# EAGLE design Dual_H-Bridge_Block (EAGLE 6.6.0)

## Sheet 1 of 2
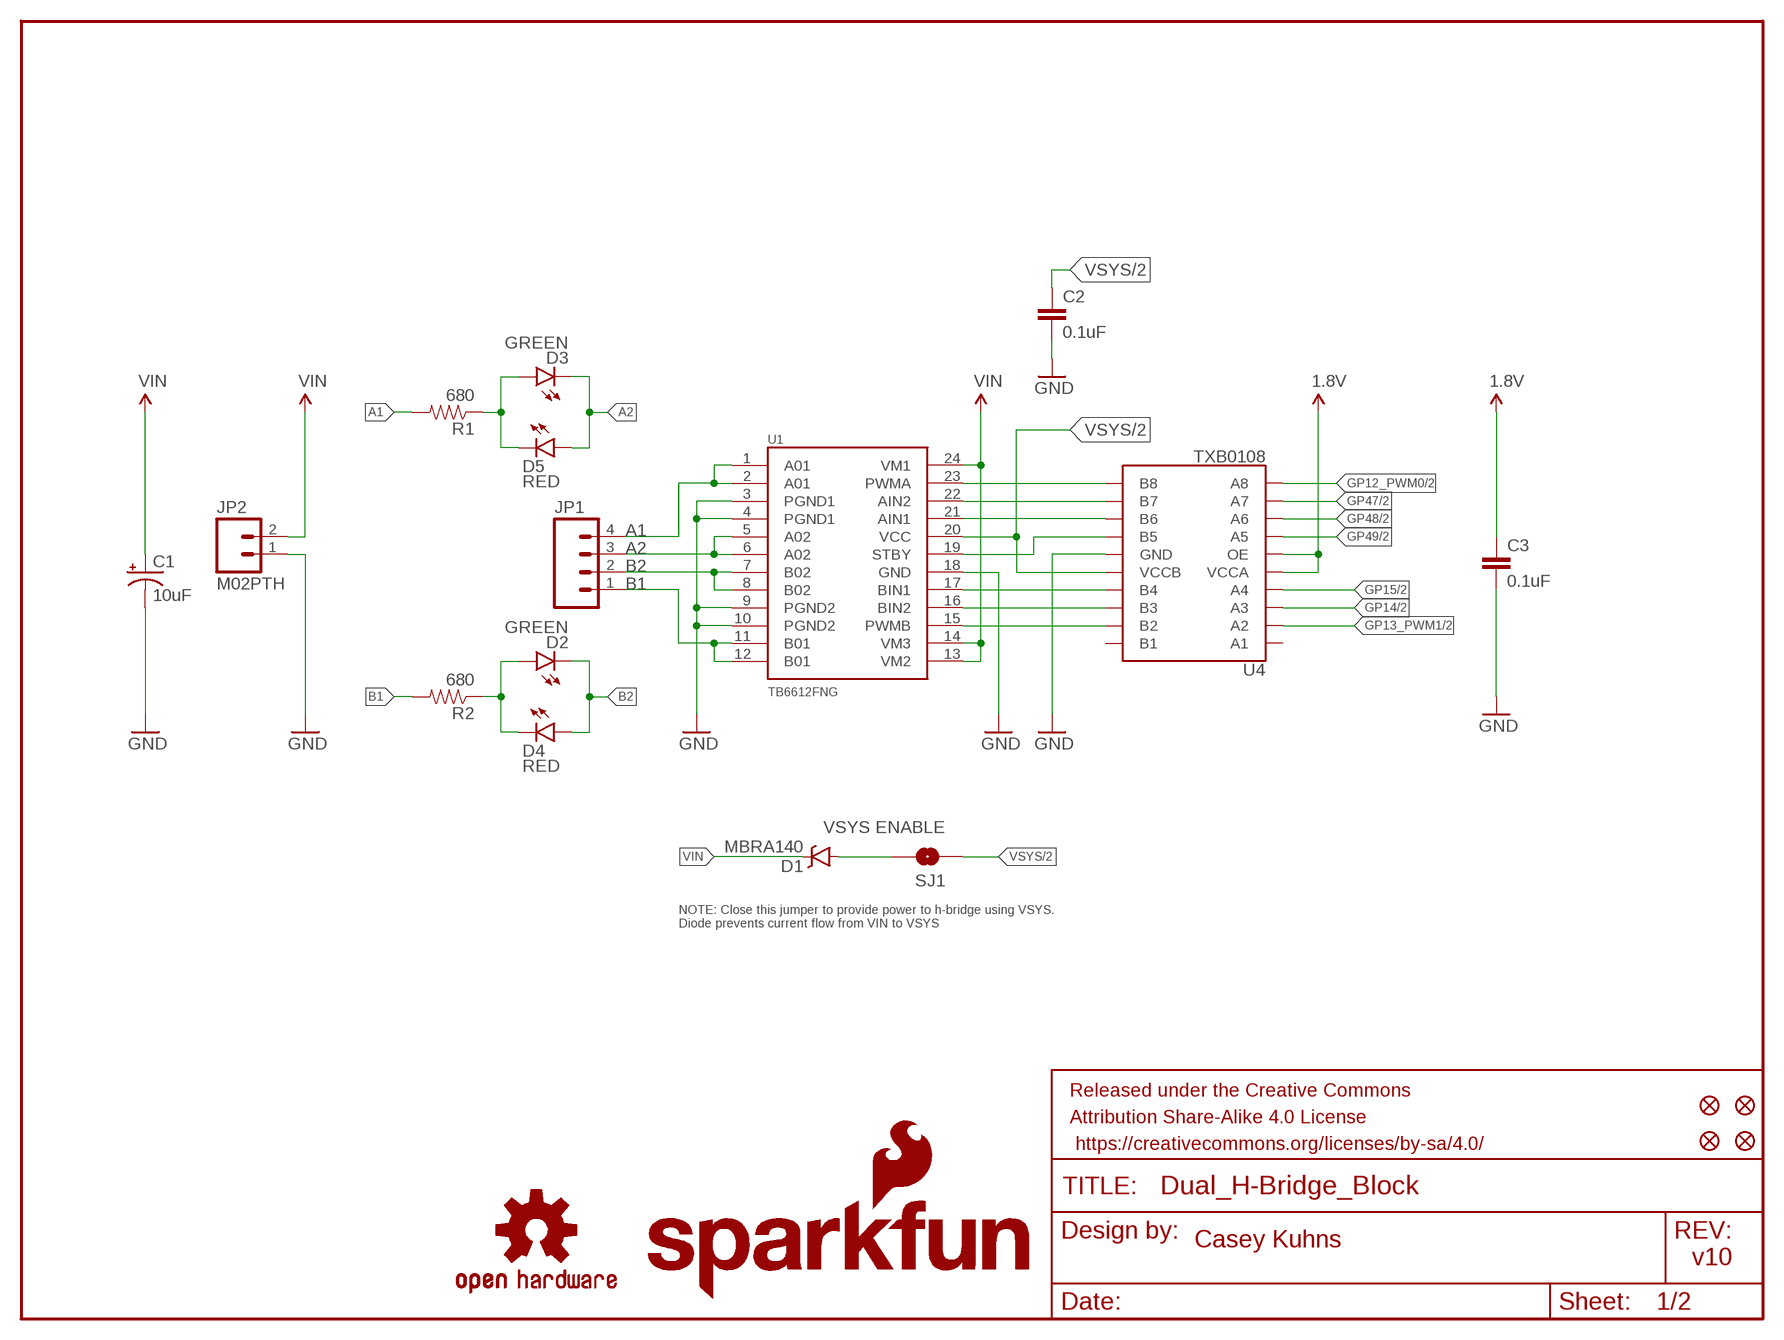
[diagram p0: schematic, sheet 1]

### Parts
C1  10uF  10UF-16V-10%(TANT)  [EIA3216]
C2  0.1uF  0.1UF-25V(+80/-20%)(0603)  [0603-CAP]
C3  0.1uF  0.1UF-25V(+80/-20%)(0603)  [0603-CAP]
D1  MBRA140  DIODE-SCHOTTKY-MBRA140  [SMA-DIODE]
D2  GREEN  LED-GREEN0603  [LED-0603]
D3  GREEN  LED-GREEN0603  [LED-0603]
D4  RED  LED-RED0603  [LED-0603]
D5  RED  LED-RED0603  [LED-0603]
FID1  FIDUCIAL1X2  [FIDUCIAL-1X2]
FID2  FIDUCIAL1X2  [FIDUCIAL-1X2]
FID3  FIDUCIAL1X2  [FIDUCIAL-1X2]
FID4  FIDUCIAL1X2  [FIDUCIAL-1X2]
FRAME1  FRAME-LETTER  [CREATIVE_COMMONS]
JP1  M04PTH  [1X04]
JP2  M02PTH  [1X02]
LOGO1  OSHW-LOGOS  [OSHW-LOGO-S]
LOGO4  SFE_LOGO_NAME_FLAME.1_INCH  [SFE_LOGO_NAME_FLAME_.1]
R1  680  680OHM1/10W5%(0603)  [0603-RES]
R2  680  680OHM1/10W5%(0603)  [0603-RES]
SJ1  VSYS ENABLE  JUMPER-PAD-2-NOYES_SILK  [PAD-JUMPER-2-NO_YES_SILK]
U1  TB6612FNG  TB6621FNG  [SSOP24]
U4  TXB0108  [UFDFN-20]

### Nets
1.8V: C3.1 U4.5(VCCA) U4.6(OE) ; also sheet 2
A1: JP1.4 R1.2 U1.1(A01) U1.2(A01)
A2: D3.C D5.A JP1.3 U1.5(A02) U1.6(A02)
B1: JP1.1 R2.2 U1.11(B01) U1.12(B01)
B2: D2.C D4.A JP1.2 U1.7(B02) U1.8(B02)
GND: C1.C(-) C2.2 C3.2 JP2.1 U1.3(PGND1) U1.4(PGND1) U1.9(PGND2) U1.10(PGND2) U1.18(GND) U4.15(GND) ; also sheet 2
GP12_PWM0: U4.10(A8) ; also sheet 2
GP13_PWM1: U4.2(A2) ; also sheet 2
GP14: U4.3(A3) ; also sheet 2
GP15: U4.4(A4) ; also sheet 2
GP47: U4.9(A7) ; also sheet 2
GP48: U4.8(A6) ; also sheet 2
GP49: U4.7(A5) ; also sheet 2
N$1: D1.A SJ1.2
N$2: D2.A D4.C R2.1
N$3: U1.15(PWMB) U4.19(B2)
N$4: U1.23(PWMA) U4.11(B8)
N$5: D3.A D5.C R1.1
N$10: U1.19(STBY) U4.14(B5)
N$11: U1.17(BIN1) U4.17(B4)
N$12: U1.16(BIN2) U4.18(B3)
N$14: U1.21(AIN1) U4.13(B6)
N$15: U1.22(AIN2) U4.12(B7)
VIN: C1.A(+) D1.C JP2.2 U1.13(VM2) U1.14(VM3) U1.24(VM1)
VSYS: C2.1 SJ1.1 U1.20(VCC) U4.16(VCCB) ; also sheet 2
Unconnected: U4.1(A1) U4.20(B1)

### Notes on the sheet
- NOTE: Close this jumper to provide power to h-bridge using VSYS.
  Diode prevents current flow from VIN to VSYS
- Casey Kuhns
- v10

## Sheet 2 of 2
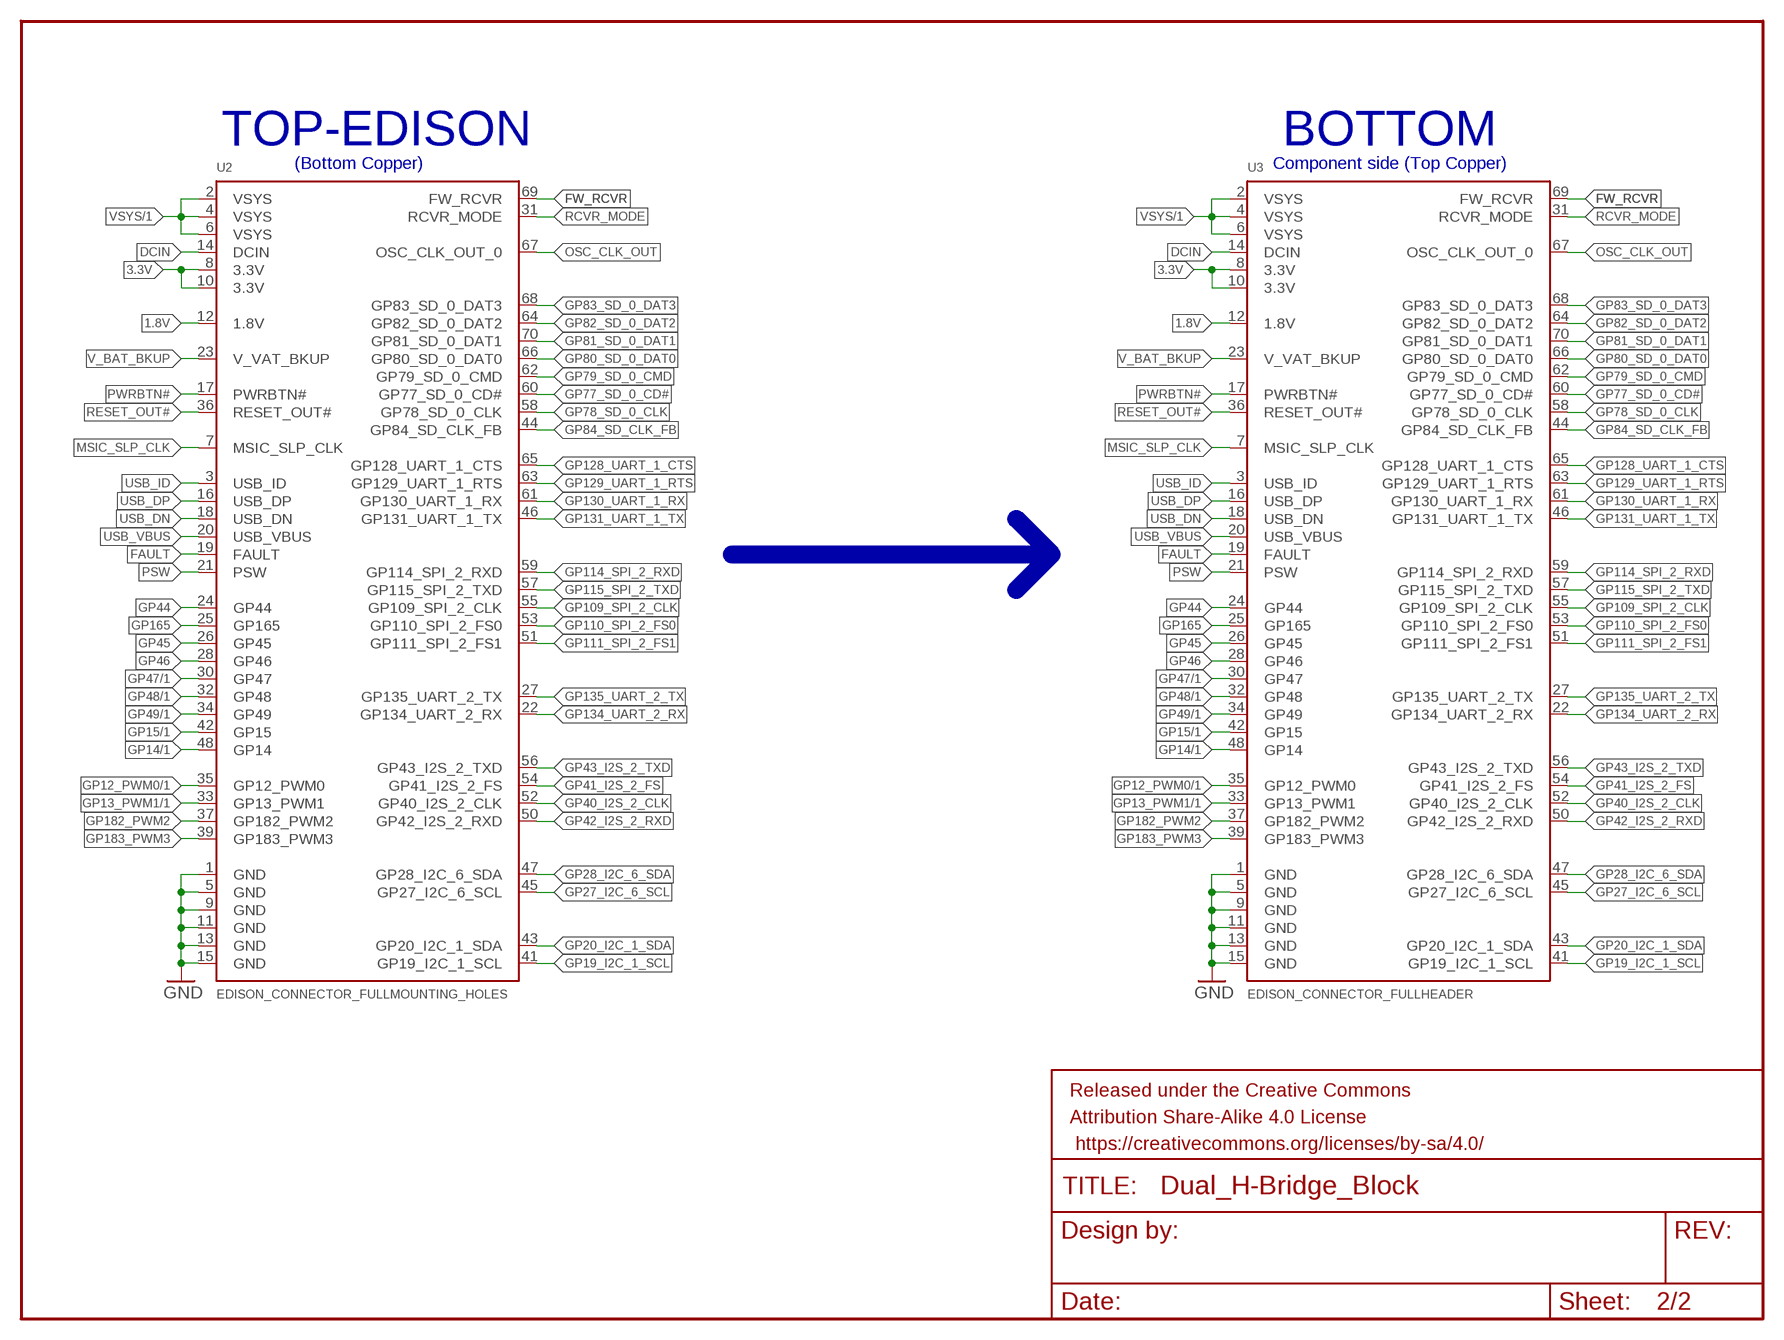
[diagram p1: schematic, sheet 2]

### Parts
FRAME2  FRAME-LETTER  [CREATIVE_COMMONS]
U2  EDISON_CONNECTOR_FULLMOUNTING_HOLES  [EDISON_DAUGHTER]
U3  EDISON_CONNECTOR_FULLHEADER  [DF40C-70DP-0.4(51)]

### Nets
1.8V: U2.12(1.8V) U3.12(1.8V) ; also sheet 1
3.3V: U2.8(3.3V) U2.10(3.3V) U3.8(3.3V) U3.10(3.3V)
DCIN: U2.14(DCIN) U3.14(DCIN)
FAULT: U2.19(FAULT) U3.19(FAULT)
FW_RCVR: U2.69(FW_RCVR) U3.69(FW_RCVR)
GND: U2.1(GND) U2.5(GND) U2.9(GND) U2.11(GND) U2.13(GND) U2.15(GND) U3.1(GND) U3.5(GND) U3.9(GND) U3.11(GND) U3.13(GND) U3.15(GND) ; also sheet 1
GP12_PWM0: U2.35(GP12_PWM0) U3.35(GP12_PWM0) ; also sheet 1
GP13_PWM1: U2.33(GP13_PWM1) U3.33(GP13_PWM1) ; also sheet 1
GP14: U2.48(GP14) U3.48(GP14) ; also sheet 1
GP15: U2.42(GP15) U3.42(GP15) ; also sheet 1
GP19_I2C_1_SCL: U2.41(GP19_I2C_1_SCL) U3.41(GP19_I2C_1_SCL)
GP20_I2C_1_SDA: U2.43(GP20_I2C_1_SDA) U3.43(GP20_I2C_1_SDA)
GP27_I2C_6_SCL: U2.45(GP27_I2C_6_SCL) U3.45(GP27_I2C_6_SCL)
GP28_I2C_6_SDA: U2.47(GP28_I2C_6_SDA) U3.47(GP28_I2C_6_SDA)
GP40_I2S_2_CLK: U2.52(GP40_I2S_2_CLK) U3.52(GP40_I2S_2_CLK)
GP41_I2S_2_FS: U2.54(GP41_I2S_2_FS) U3.54(GP41_I2S_2_FS)
GP42_I2S_2_RXD: U2.50(GP42_I2S_2_RXD) U3.50(GP42_I2S_2_RXD)
GP43_I2S_2_TXD: U2.56(GP43_I2S_2_TXD) U3.56(GP43_I2S_2_TXD)
GP44: U2.24(GP44) U3.24(GP44)
GP45: U2.26(GP45) U3.26(GP45)
GP46: U2.28(GP46) U3.28(GP46)
GP47: U2.30(GP47) U3.30(GP47) ; also sheet 1
GP48: U2.32(GP48) U3.32(GP48) ; also sheet 1
GP49: U2.34(GP49) U3.34(GP49) ; also sheet 1
GP77_SD_0_CD#: U2.60(GP77_SD_0_CD#) U3.60(GP77_SD_0_CD#)
GP78_SD_0_CLK: U2.58(GP78_SD_0_CLK) U3.58(GP78_SD_0_CLK)
GP79_SD_0_CMD: U2.62(GP79_SD_0_CMD) U3.62(GP79_SD_0_CMD)
GP80_SD_0_DAT0: U2.66(GP80_SD_0_DAT0) U3.66(GP80_SD_0_DAT0)
GP81_SD_0_DAT1: U2.70(GP81_SD_0_DAT1) U3.70(GP81_SD_0_DAT1)
GP82_SD_0_DAT2: U2.64(GP82_SD_0_DAT2) U3.64(GP82_SD_0_DAT2)
GP83_SD_0_DAT3: U2.68(GP83_SD_0_DAT3) U3.68(GP83_SD_0_DAT3)
GP84_SD_CLK_FB: U2.44(GP84_SD_CLK_FB) U3.44(GP84_SD_CLK_FB)
GP109_SPI_2_CLK: U2.55(GP109_SPI_2_CLK) U3.55(GP109_SPI_2_CLK)
GP110_SPI_2_FS0: U2.53(GP110_SPI_2_FS0) U3.53(GP110_SPI_2_FS0)
GP111_SPI_2_FS1: U2.51(GP111_SPI_2_FS1) U3.51(GP111_SPI_2_FS1)
GP114_SPI_2_RXD: U2.59(GP114_SPI_2_RXD) U3.59(GP114_SPI_2_RXD)
GP115_SPI_2_TXD: U2.57(GP115_SPI_2_TXD) U3.57(GP115_SPI_2_TXD)
GP128_UART_1_CTS: U2.65(GP128_UART_1_CTS) U3.65(GP128_UART_1_CTS)
GP129_UART_1_RTS: U2.63(GP129_UART_1_RTS) U3.63(GP129_UART_1_RTS)
GP130_UART_1_RX: U2.61(GP130_UART_1_RX) U3.61(GP130_UART_1_RX)
GP131_UART_1_TX: U2.46(GP131_UART_1_TX) U3.46(GP131_UART_1_TX)
GP134_UART_2_RX: U2.22(GP134_UART_2_RX) U3.22(GP134_UART_2_RX)
GP135_UART_2_TX: U2.27(GP135_UART_2_TX) U3.27(GP135_UART_2_TX)
GP165: U2.25(GP165) U3.25(GP165)
GP182_PWM2: U2.37(GP182_PWM2) U3.37(GP182_PWM2)
GP183_PWM3: U2.39(GP183_PWM3) U3.39(GP183_PWM3)
MSIC_SLP_CLK: U2.7(MSIC_SLP_CLK) U3.7(MSIC_SLP_CLK)
OSC_CLK_OUT: U2.67(OSC_CLK_OUT_0) U3.67(OSC_CLK_OUT_0)
PSW: U2.21(PSW) U3.21(PSW)
PWRBTN#: U2.17(PWRBTN#) U3.17(PWRBTN#)
RCVR_MODE: U2.31(RCVR_MODE) U3.31(RCVR_MODE)
RESET_OUT#: U2.36(RESET_OUT#) U3.36(RESET_OUT#)
USB_DN: U2.18(USB_DN) U3.18(USB_DN)
USB_DP: U2.16(USB_DP) U3.16(USB_DP)
USB_ID: U2.3(USB_ID) U3.3(USB_ID)
USB_VBUS: U2.20(USB_VBUS) U3.20(USB_VBUS)
V_BAT_BKUP: U2.23(V_VAT_BKUP) U3.23(V_VAT_BKUP)
VSYS: U2.2(VSYS) U2.4(VSYS) U2.6(VSYS) U3.2(VSYS) U3.4(VSYS) U3.6(VSYS) ; also sheet 1

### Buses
B$1

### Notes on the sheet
- TOP-EDISON | BOTTOM
- (Bottom Copper) | Component side (Top Copper)

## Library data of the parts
C1 = SparkFun-Capacitors:10UF-16V-10%(TANT): CAP-00811; PROD_ID: CAP-00811
C2 C3 = SparkFun-Capacitors:0.1UF-25V(+80/-20%)(0603): CAP-00810; PROD_ID: CAP-00810
D1 = SparkFun-DiscreteSemi:DIODE-SCHOTTKY: Schottky diodes in SFE's production catalog; PROD_ID: DIO-08053
D2 D3 = SparkFun-LED:LED-GREEN: Various green LEDs; PROD_ID: DIO-00821
D4 D5 = SparkFun-LED:LED-RED: Assorted Red LEDs; PROD_ID: DIO-00819
FID1-FID4 = SparkFun-Aesthetics:FIDUCIAL: Fiducial Alignment Points
FRAME1 FRAME2 = SparkFun-Aesthetics:FRAME-LETTER: Schematic Frame
JP1 = SparkFun-Connectors:M04: Header 4 Standard 4-pin 0.1" header. Use with straight break away headers (SKU : PRT-00116), right angle break away headers (PRT-00553), swiss pins (PRT-00743), machine pins (PRT-00117), and female headers (PRT-00115). Molex polarized connector foot print use with SKU : PRT-08231 with associated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
JP2 = SparkFun-Connectors:M02: Standard 2-pin 0.1" header. Use with
LOGO1 = SparkFun-Aesthetics:OSHW-LOGO: Open Source Hardware Logo This logo indicates the piece of hardware it is found on incorporates a OSHW license and/or adheres to the definition of open source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
LOGO4 = SparkFun-Aesthetics:SFE_LOGO_NAME_FLAME: SFE Logo, name and flame
R1 R2 = SparkFun-Resistors:680OHM1/10W5%(0603): RES-09333; PROD_ID: RES-09333
SJ1 = SparkFun-Passives:JUMPER-PAD-2-NO
U1 = SparkFun-PowerIC:TB6621FNG: Toshiba 1A dual motor driver IC-09363; PROD_ID: IC-09363
U2 U3 = Edison:EDISON_CONNECTOR_FULL
U4 = Testing:TXB0108; PROD_ID: IC-12292

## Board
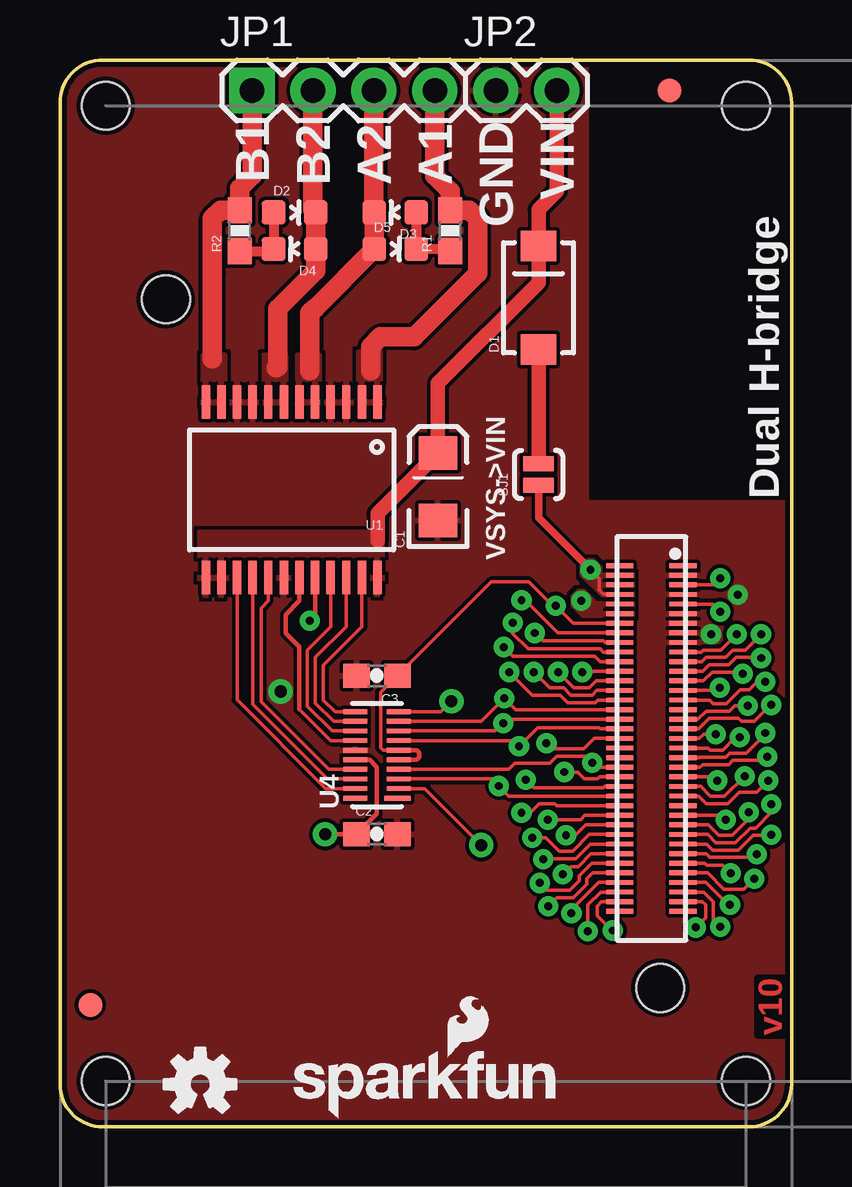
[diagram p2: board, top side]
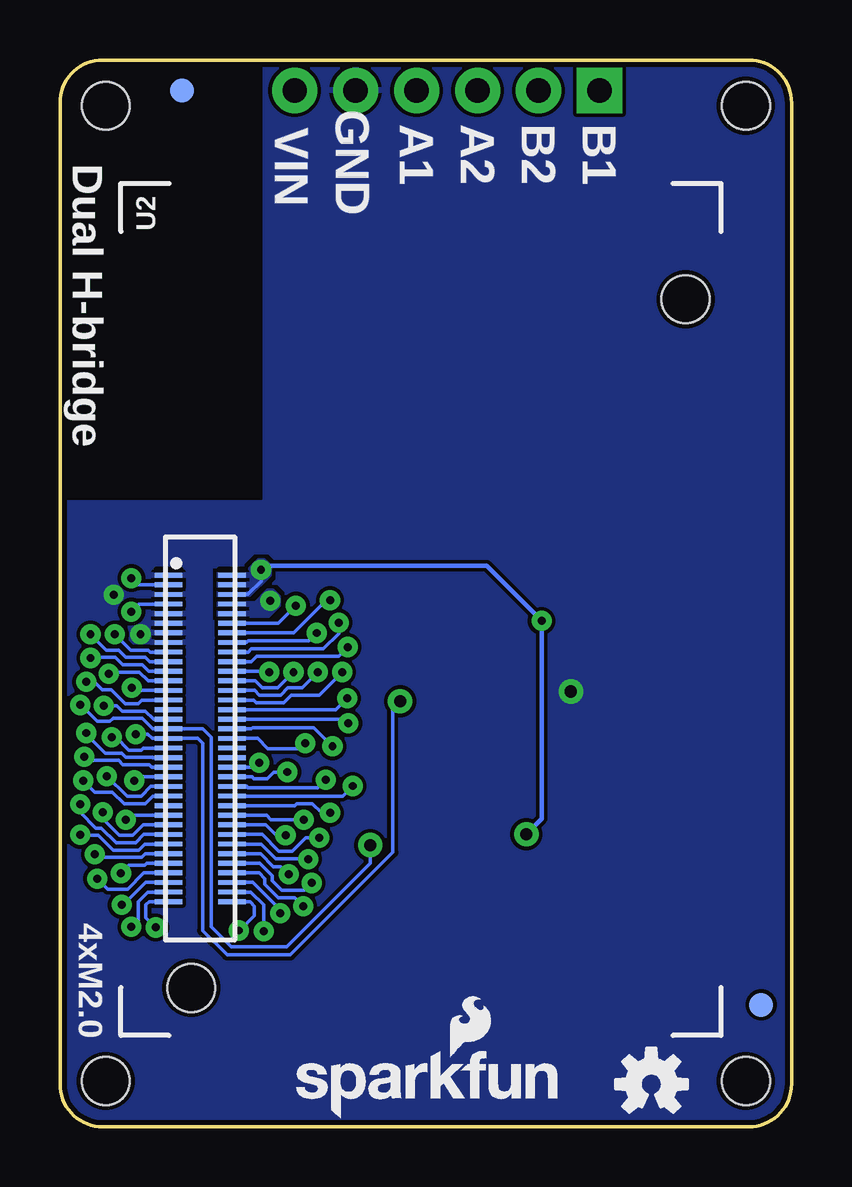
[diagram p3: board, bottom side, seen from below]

Size 30.48 x 44.45 mm. Coordinates in mm from the lower left corner, seen from the top.
Outline: 30.48,42.67 30.48,1.78 arc-90 28.7,0 1.78,0 arc-90 0,1.78 0,42.67 arc-90 1.78,44.45 28.7,44.45 arc-90 30.48,42.67
Copper layers (1*16): Top 0.035mm / dielectric 1.5mm / Bottom 0.035mm
Design rules "SparkFun-2-layer *": minimum track width 6mil, minimum drill 13mil, track to track 6mil, track to pad 6mil, pad to pad 6mil, via to via 6mil, smd to smd 6mil, copper to edge 8mil, drill to drill 8mil, minimum pad ring 12mil, minimum via ring 10mil, stop-mask expansion 4mil, vias tented up to drill 20mil, thermal gap 6mil
Holes 2 mm at 28.57,1.91 1.91,1.91 1.91,42.55 28.57,42.55
tRestrict: area 22.1,26.2 to 30.5,44.5
bRestrict: area 22.1,26.2 to 30.5,44.5; 2 lines

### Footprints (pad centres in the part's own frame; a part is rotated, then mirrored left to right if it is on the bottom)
EIA3216 = smd 1.4 x 1.6: A 1.4,0; C -1.4,0
0603-CAP = smd 1.1 x 1: 1 -0.85,0; 2 0.85,0
SMA-DIODE = smd 1.27 x 1.47: A -2.15,0; C 2.15,0
LED-0603 = smd 1 x 1: A 0,-0.877; C 0,0.877
FIDUCIAL-1X2 = smd 1 x 1: 1 0,0
1X04 = drill 1.016 pad 1.88 square: 1 0,0 | drill 1.016 pad 1.88: 2 2.54,0; 3 5.08,0; 4 7.62,0
1X02 = drill 1.016 pad 1.88: 1 0,0; 2 2.54,0
0603-RES = smd 1.1 x 1: 1 -0.85,0; 2 0.85,0
PAD-JUMPER-2-NO_YES_SILK = smd 0.635 x 1.27: 1 -0.45,0; 2 0.45,0
SSOP24 = smd 0.348 x 1.397: 1 -3.575,-3.656; 2 -2.925,-3.656; 3 -2.275,-3.656; 4 -1.625,-3.656; 5 -0.975,-3.656; 6 -0.325,-3.656; 7 0.325,-3.656; 8 0.975,-3.656; 9 1.625,-3.656; 10 2.275,-3.656; 11 2.925,-3.656; 12 3.575,-3.656; 13 3.575,3.656; 14 2.925,3.656; 15 2.275,3.656; 16 1.625,3.656; 17 0.975,3.656; 18 0.325,3.656; 19 -0.325,3.656; 20 -0.975,3.656; 21 -1.625,3.656; 22 -2.275,3.656; 23 -2.925,3.656; 24 -3.575,3.656
EDISON_DAUGHTER = smd 1.14 x 0.2: 1 1.98,19.17; 2 4.62,19.17; 3 1.98,18.77; 4 4.62,18.77; 5 1.98,18.37; 6 4.62,18.37; 7 1.98,17.97; 8 4.62,17.97; 9 1.98,17.57; 10 4.62,17.57; 11 1.98,17.17; 12 4.62,17.17; 13 1.98,16.77; 14 4.62,16.77; 15 1.98,16.37; 16 4.62,16.37; 17 1.98,15.97; 18 4.62,15.97; 19 1.98,15.57; 20 4.62,15.57; 21 1.98,15.17; 22 4.62,15.17; 23 1.98,14.77; 24 4.62,14.77; 25 1.98,14.37; 26 4.62,14.37; 27 1.98,13.97; 28 4.62,13.97; 29 1.98,13.57; 30 4.62,13.57; 31 1.98,13.17; 32 4.62,13.17; 33 1.98,12.77; 34 4.62,12.77; 35 1.98,12.37; 36 4.62,12.37; 37 1.98,11.97; 38 4.62,11.97; 39 1.98,11.57; 40 4.62,11.57; 41 1.98,11.17; 42 4.62,11.17; 43 1.98,10.77; 44 4.62,10.77; 45 1.98,10.37; 46 4.62,10.37; 47 1.98,9.97; 48 4.62,9.97; 49 1.98,9.57; 50 4.62,9.57; 51 1.98,9.17; 52 4.62,9.17; 53 1.98,8.77; 54 4.62,8.77; 55 1.98,8.37; 56 4.62,8.37; 57 1.98,7.97; 58 4.62,7.97; 59 1.98,7.57; 60 4.62,7.57; 61 1.98,7.17; 62 4.62,7.17; 63 1.98,6.77; 64 4.62,6.77; 65 1.98,6.37; 66 4.62,6.37; 67 1.98,5.97; 68 4.62,5.97; 69 1.98,5.57; 70 4.62,5.57 | hole 2: 23.53,30.67; 2.93,1.98
DF40C-70DP-0.4(51) = smd 0.2 x 1.14 bottom: 1 6.8,1.32; 2 6.8,-1.32; 3 6.4,1.32; 4 6.4,-1.32; 5 6,1.32; 6 6,-1.32; 7 5.6,1.32; 8 5.6,-1.32; 9 5.2,1.32; 10 5.2,-1.32; 11 4.8,1.32; 12 4.8,-1.32; 13 4.4,1.32; 14 4.4,-1.32; 15 4,1.32; 16 4,-1.32; 17 3.6,1.32; 18 3.6,-1.32; 19 3.2,1.32; 20 3.2,-1.32; 21 2.8,1.32; 22 2.8,-1.32; 23 2.4,1.32; 24 2.4,-1.32; 25 2,1.32; 26 2,-1.32; 27 1.6,1.32; 28 1.6,-1.32; 29 1.2,1.32; 30 1.2,-1.32; 31 0.8,1.32; 32 0.8,-1.32; 33 0.4,1.32; 34 0.4,-1.32; 35 0,1.32; 36 0,-1.32; 37 -0.4,1.32; 38 -0.4,-1.32; 39 -0.8,1.32; 40 -0.8,-1.32; 41 -1.2,1.32; 42 -1.2,-1.32; 43 -1.6,1.32; 44 -1.6,-1.32; 45 -2,1.32; 46 -2,-1.32; 47 -2.4,1.32; 48 -2.4,-1.32; 49 -2.8,1.32; 50 -2.8,-1.32; 51 -3.2,1.32; 52 -3.2,-1.32; 53 -3.6,1.32; 54 -3.6,-1.32; 55 -4,1.32; 56 -4,-1.32; 57 -4.4,1.32; 58 -4.4,-1.32; 59 -4.8,1.32; 60 -4.8,-1.32; 61 -5.2,1.32; 62 -5.2,-1.32; 63 -5.6,1.32; 64 -5.6,-1.32; 65 -6,1.32; 66 -6,-1.32; 67 -6.4,1.32; 68 -6.4,-1.32; 69 -6.8,1.32; 70 -6.8,-1.32; NC1 7.2,1.32; NC2 7.2,-1.32; NC3 -7.2,-1.32; NC4 -7.2,1.32
UFDFN-20 = smd 0.2 x 1.1: 1 -1.8,-0.85 | smd 0.2 x 1: 2 -1.4,-0.9; 3 -1,-0.9; 4 -0.6,-0.9; 5 -0.2,-0.9; 6 0.2,-0.9; 7 0.6,-0.9; 8 1,-0.9; 9 1.4,-0.9; 10 1.8,-0.9; 11 1.8,0.9; 12 1.4,0.9; 13 1,0.9; 14 0.6,0.9; 15 0.2,0.9; 16 -0.2,0.9; 17 -0.6,0.9; 18 -1,0.9; 19 -1.4,0.9; 20 -1.8,0.9

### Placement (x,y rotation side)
C1  15.75,26.67 90 top
C2  13.21,12.19 0 top
C3  13.21,18.8 180 top
D1  19.94,34.54 90 top
D2  9.78,38.1 270 top
D3  13.97,38.1 90 top
D4  9.78,36.58 90 top
D5  13.97,36.58 270 top
FID1  1.27,5.08 0 top
FID2  25.4,43.18 0 top
FID3  1.27,5.08 0 bottom
FID4  25.4,43.18 0 bottom
FRAME1  not placed on the board
FRAME2  not placed on the board
JP1  8,43.18 0 top
JP2  18.16,43.18 0 top
LOGO1  5.84,1.78 0 top
LOGO2  OSHW-LOGOS  [OSHW-LOGO-S]  5.84,1.78 0 bottom
LOGO3  SFE_LOGO_NAME_FLAME.1_INCH  [SFE_LOGO_NAME_FLAME_.1]  21.08,0.25 0 bottom
LOGO4  9.3,0.25 0 top
R1  16.26,37.34 90 top
R2  7.49,37.34 90 top
SJ1  19.94,27.18 90 top
U1  9.65,26.54 180 top
U2  27.94,3.81 0 bottom
U3  24.64,16.18 90 bottom
U4  13.21,15.49 90 top

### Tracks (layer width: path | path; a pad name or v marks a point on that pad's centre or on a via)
1.8V  (via drill 0.33)
  Top 0.152: U3.12 21.39,20.98 v20.65,21.72 20.52,21.72 19.53,22.71 17.97,22.71 C3.1 13.36,18.1 13.36,15.8 13.46,15.69 U4.6
  Top 0.178: U4.5 14.86,15.29 14.96,15.39 14.96,15.6 14.86,15.7 U4.6
  Bottom 0.152: U3.12 21.39,20.98 v20.65,21.72
3.3V  (via drill 0.33)
  Bottom 0.152: U3.10
  other vias: 21.72,21.92
  pour Bottom (isolate 0.051): 21.59,22.35 21.84,22.35 22.35,21.84 23.88,21.84 23.88,21.21 21.84,21.21 21.34,21.72 21.34,22.1
  pour Top (isolate 0.051): 21.59,22.35 21.84,22.35 22.35,21.84 23.88,21.84 23.88,21.21 21.84,21.21 21.34,21.72 21.34,22.1
A1
  Top 0.813: JP1.4 15.62,39.62 16.26,38.99 R1.2 17.06,38.19 17.4,37.85 17.4,35.56 14.75,32.91 13.35,32.91 12.95,32.51 12.95,31.5
  pour Top (isolate 0.305): 12.45,30.1 13.34,30.1 13.34,32.26 12.45,32.26
A2
  Top 0.406: 13.08,38.11 D3.C
  Top 0.813: D3.C D5.A 10.63,34.11 10.62,34.11 10.41,33.91 10.41,31.5 | JP1.3 13.08,38.11
  pour Top (isolate 0.254): 9.91,30.1 10.79,30.1 10.79,32.13 9.91,32.13
B1
  Top 0.254: 6.48,31.88 6.35,32.01
  Top 0.813: JP1.1 8,39.62 7.49,39.12 R2.2 6.69,38.19 6.35,37.85 6.35,35.56 6.35,32.01
  pour Top (isolate 0.305): 5.97,30.1 6.86,30.1 6.86,32.13 5.97,32.13
B2
  Top 0.406: 10.54,38.22 D2.C
  Top 0.813: D2.C D4.A 10.66,35.67 9.07,34.09 9.07,31.68 9.02,31.62 | JP1.2 10.54,38.22
  pour Top (isolate 0.254): 8.51,30.1 9.4,30.1 9.4,32.13 8.51,32.13
DCIN  (via drill 0.33)
  Top 0.152: U3.14 20.75,20.58 19.38,21.95 v19.23,21.95
  Bottom 0.152: v19.23,21.95 19.38,21.95 20.75,20.58 U3.14
FAULT  (via drill 0.33)
  Top 0.152: U3.19 26.75,19.38 26.92,19.56 27.74,19.56 28.04,19.86 28.55,19.86 v29.21,20.52
  Bottom 0.152: v29.21,20.52 28.55,19.86 28.04,19.86 27.74,19.56 26.92,19.56 26.75,19.38 U3.19
FW_RCVR  (via drill 0.33)
  Top 0.152: v26.49,8.31 26.9,8.71 26.9,9.25 26.76,9.38 U3.69
  Bottom 0.152: U3.69 26.76,9.38 26.9,9.25 26.9,8.71 v26.49,8.31
GND  (via drill 0.33, 0.51)
  other vias: 27.13,20.52 28.24,22.17 9.19,18.14
  pour Bottom (isolate 0.051, rank 6): 30.48,42.67 30.48,1.78 arc-90 28.7,0 1.78,0 arc-90 0,1.78 0,42.67 arc-90 1.78,44.45 28.7,44.45 arc-90
  pour Top (isolate 0.051, rank 6): 30.48,1.73 arc-90 28.75,0 1.78,0 arc-90 0,1.78 0,42.67 arc-90 1.78,44.45 28.7,44.45 arc-90 30.48,42.67
GP12_PWM0  (via drill 0.33, 0.51)
  Top 0.152: U3.35 26.64,16.18 26.82,16.36 v27.33,16.36 | U4.10 15.87,17.29 v16.31,17.73
  Bottom 0.152: v27.33,16.36 26.82,16.36 26.64,16.18 U3.35 | U3.35 | U3.35 24.74,16.18 24.54,15.98 24.54,8.18 23.52,7.16 20.88,7.16 16.61,11.43 16.61,17.42 v16.31,17.73
GP13_PWM1  (via drill 0.33, 0.51)
  Top 0.152: v29.64,17.58 29.62,17.58 28.93,16.89 28.4,16.89 28.27,17.02 27.05,17.02 26.61,16.58 U3.33 | v17.55,11.73 15.19,14.09 U4.2
  Bottom 0.152: v29.64,17.58 29.62,17.58 28.93,16.89 28.4,16.89 28.27,17.02 27.05,17.02 26.61,16.58 U3.33 24.53,16.58 24.18,16.23 24.18,8.33 23.34,7.49 21.03,7.49 17.55,10.97 v17.55,11.73
GP14  (via drill 0.33)
  Top 0.152: U3.48 18.71,13.78 v18.29,14.2 17.99,14.49 U4.3
  Bottom 0.152: v18.29,14.2 18.71,13.78 U3.48
GP15  (via drill 0.33)
  Top 0.152: U3.42 22.36,14.98 v22.17,15.16 21.89,15.44 20.7,15.44 20.4,15.14 18.95,15.14 18.7,14.89 U4.4
  Bottom 0.152: v22.17,15.16 22.36,14.98 U3.42
GP19_I2C_1_SCL  (via drill 0.33)
  Top 0.152: U3.41 26.66,14.98 26.77,15.09 27.86,15.09 28.04,15.27 29.31,15.27 v29.46,15.42
  Bottom 0.152: v29.46,15.42 29.31,15.27 28.04,15.27 27.86,15.09 26.77,15.09 26.66,14.98 U3.41
GP20_I2C_1_SDA  (via drill 0.33)
  Top 0.152: U3.43 27.23,14.58 v27.38,14.43
  Bottom 0.152: v27.38,14.43 27.23,14.58 U3.43 | U3.43
GP27_I2C_6_SCL  (via drill 0.33)
  Top 0.152: v28.52,14.61 27.69,13.77 27.1,13.77 26.69,14.18 U3.45
  Bottom 0.152: U3.45 26.69,14.18 27.1,13.77 27.69,13.77 v28.52,14.61
GP28_I2C_6_SDA  (via drill 0.33)
  Top 0.152: U3.47 26.61,13.78 26.92,13.46 27.81,13.46 28.3,13.95 29.03,13.95 v29.52,14.43
  Bottom 0.152: v29.52,14.43 29.03,13.95 28.3,13.95 27.81,13.46 26.92,13.46 26.61,13.78 U3.47
GP40_I2S_2_CLK  (via drill 0.33)
  Top 0.152: U3.52 21.87,12.98 21.69,12.8 v20.32,12.8
  Bottom 0.152: v20.32,12.8 21.69,12.8 21.87,12.98 U3.52
GP41_I2S_2_FS  (via drill 0.33)
  Top 0.152: v21.08,12.14 21.46,12.14 21.9,12.58 U3.54
  Bottom 0.152: U3.54 21.9,12.58 21.46,12.14 v21.08,12.14
GP42_I2S_2_RXD  (via drill 0.33)
  Top 0.152: v19.23,13.08 19.58,13.08 19.96,13.46 20.62,13.46 20.71,13.38 U3.50
  Bottom 0.152: v19.23,13.08 19.58,13.08 19.96,13.46 20.62,13.46 20.71,13.38 U3.50
GP43_I2S_2_TXD  (via drill 0.33)
  Top 0.152: U3.56 22.06,12.18 21.36,11.48 20.8,11.48 20.24,12.04 v19.68,12.04
  Bottom 0.152: v19.68,12.04 20.24,12.04 20.8,11.48 21.36,11.48 22.06,12.18 U3.56
GP44  (via drill 0.33)
  Top 0.152: U3.24 22.34,18.58 22.05,18.29 21.41,18.29 v20.75,18.95
  Bottom 0.152: v20.75,18.95 21.41,18.29 22.05,18.29 22.34,18.58 U3.24
GP45  (via drill 0.33)
  Top 0.152: v19.74,18.95 20.4,18.29 20.98,18.29 21.29,17.98 22.17,17.98 22.37,18.18 U3.26
  Bottom 0.152: U3.26 22.37,18.18 22.17,17.98 21.29,17.98 20.98,18.29 20.4,18.29 v19.74,18.95
GP46  (via drill 0.33)
  Top 0.152: U3.28 22.4,17.78 22.3,17.68 21.16,17.68 20.85,17.98 19.68,17.98 v18.72,18.95
  Bottom 0.152: U3.28 22.4,17.78 22.3,17.68 21.16,17.68 20.85,17.98 19.68,17.98 v18.72,18.95
GP47  (via drill 0.33)
  Top 0.152: U3.30 22.43,17.38 22.43,17.37 19,17.37 v18.52,17.86 17.55,16.89 U4.9
  Bottom 0.152: U3.30 22.43,17.38 22.43,17.37 19,17.37 v18.52,17.86
GP48  (via drill 0.33)
  Top 0.152: U3.32 18.63,16.98 v18.47,16.82 18.14,16.49 U4.8
  Bottom 0.152: U3.32 18.63,16.98 v18.47,16.82
GP49  (via drill 0.33)
  Top 0.152: U4.7 18.88,16.09 v19.13,15.85 19.91,16.64 22.45,16.64 22.51,16.58 U3.34
  Bottom 0.152: v19.13,15.85 19.91,16.64 22.45,16.64 22.5,16.58 U3.34 | U3.34
GP77_SD_0_CD#  (via drill 0.33)
  Top 0.152: U3.60 22.12,11.38 21.59,10.85 21.29,10.85 v20.95,10.52
  Bottom 0.152: v20.95,10.52 21.29,10.85 21.59,10.85 22.12,11.38 U3.60
GP78_SD_0_CLK  (via drill 0.33)
  Top 0.152: U3.58 22.09,11.78 21.49,11.18 20.17,11.18 v20.14,11.15
  Bottom 0.152: v20.14,11.15 20.17,11.18 21.49,11.18 22.09,11.78 U3.58
GP79_SD_0_CMD  (via drill 0.33)
  Top 0.152: U3.62 22.16,10.98 21.64,10.46 21.64,10.26 21.23,9.86 20.3,9.86 v19.99,10.16
  Bottom 0.152: v19.99,10.16 20.3,9.86 21.23,9.86 21.64,10.26 21.64,10.46 22.16,10.98 U3.62
GP80_SD_0_DAT0  (via drill 0.33)
  Top 0.152: v21.31,8.89 21.31,9.04 22.45,10.18 U3.66
  Bottom 0.152: U3.66 22.45,10.18 21.31,9.04 v21.31,8.89
GP81_SD_0_DAT1  (via drill 0.33)
  Top 0.152: U3.70 22.56,9.38 22.38,9.2 22.38,8.79 22.99,8.18 v23.04,8.18
  Bottom 0.152: v23.04,8.18 22.99,8.18 22.38,8.79 22.38,9.2 22.56,9.38 U3.70
GP82_SD_0_DAT2  (via drill 0.33)
  Top 0.152: U3.64 22.19,10.58 21.95,10.34 21.95,10.11 21.39,9.55 20.7,9.55 v20.34,9.2
  Bottom 0.152: v20.34,9.2 20.7,9.55 21.39,9.55 21.95,10.11 21.95,10.34 22.19,10.58 U3.64
GP83_SD_0_DAT3  (via drill 0.33)
  Top 0.152: v22,8.15 22,9.25 22.53,9.78 U3.68
  Bottom 0.152: U3.68 22.53,9.78 22,9.25 v22,8.15
GP84_SD_CLK_FB  (via drill 0.33)
  Top 0.152: U3.44 22.48,14.58 22.4,14.5 21.84,14.5 21.57,14.78 v21.01,14.78
  Bottom 0.152: v21.01,14.78 21.57,14.78 21.84,14.5 22.4,14.5 22.48,14.58 U3.44 | U3.44
GP109_SPI_2_CLK  (via drill 0.33)
  Top 0.152: U3.55 26.99,12.18 27.33,11.84 28.14,11.84 28.75,12.45 28.98,12.45 29.64,13.11 v29.64,13.44
  Bottom 0.152: v29.64,13.44 29.64,13.11 28.98,12.45 28.75,12.45 28.14,11.84 27.33,11.84 26.99,12.18 U3.55
GP110_SPI_2_FS0  (via drill 0.33)
  Top 0.152: v28.7,13.11 28.7,12.83 28.02,12.14 27.46,12.14 27.02,12.58 U3.53
  Bottom 0.152: U3.53 27.02,12.58 27.46,12.14 28.02,12.14 28.7,12.83 v28.7,13.11
GP111_SPI_2_FS1  (via drill 0.33)
  Top 0.152: v27.74,12.8 27.56,12.98 U3.51
  Bottom 0.152: U3.51 27.56,12.98 v27.74,12.8
GP114_SPI_2_RXD  (via drill 0.33)
  Top 0.152: U3.59 26.92,11.38 27.08,11.23 28.91,11.23 v29.03,11.35
  Bottom 0.152: U3.59 26.92,11.38 27.08,11.23 28.91,11.23 v29.03,11.35
GP115_SPI_2_TXD  (via drill 0.33)
  Top 0.152: U3.57 26.95,11.78 27.2,11.53 28.27,11.53 28.88,12.14 29.62,12.14 v29.64,12.17
  Bottom 0.152: U3.57 26.95,11.78 27.2,11.53 28.27,11.53 28.88,12.14 29.62,12.14 v29.64,12.17
GP128_UART_1_CTS  (via drill 0.33)
  Top 0.152: U3.65 26.9,10.18 27.84,9.25 v27.91,9.25
  Bottom 0.152: v27.91,9.25 27.84,9.25 26.9,10.18 U3.65
GP129_UART_1_RTS  (via drill 0.33)
  Top 0.152: v28.93,10.34 28.5,9.91 27.66,9.91 26.99,10.58 U3.63
  Bottom 0.152: U3.63 26.99,10.58 27.66,9.91 28.5,9.91 v28.93,10.34
GP130_UART_1_RX  (via drill 0.33)
  Top 0.152: v27.94,10.57 27.61,10.9 26.95,10.9 26.87,10.98 U3.61
  Bottom 0.152: U3.61 26.87,10.98 26.95,10.9 27.61,10.9 v27.94,10.57
GP131_UART_1_TX  (via drill 0.33)
  Top 0.152: 19.43,14.43 v19.41,14.45 | 19.68,14.18 v19.41,14.45 | U3.46 22.69,14.18 22.63,14.12 19.74,14.12 v19.41,14.45
  Bottom 0.152: 19.43,14.43 v19.41,14.45 | 19.66,14.2 v19.41,14.45 | 19.68,14.18 v19.41,14.45 | U3.46 22.71,14.18 22.65,14.12 19.74,14.12 v19.41,14.45
GP134_UART_2_RX  (via drill 0.33)
  Top 0.152: v21.77,18.95 21.8,18.98 U3.22
  Bottom 0.152: U3.22 21.8,18.98 v21.77,18.95
GP135_UART_2_TX  (via drill 0.33)
  Top 0.152: v29.39,18.54 29.06,18.54 28.73,18.21 28.35,18.21 27.76,17.63 27.23,17.63 27.08,17.78 U3.27
  Bottom 0.152: U3.27 27.08,17.78 27.23,17.63 27.76,17.63 28.35,18.21 28.73,18.21 29.06,18.54 v29.39,18.54
GP165  (via drill 0.33)
  Top 0.152: v27.48,18.29 27.38,18.18 U3.25
  Bottom 0.152: U3.25 27.38,18.18 v27.48,18.29
GP182_PWM2  (via drill 0.33)
  Top 0.152: U3.37 27.02,15.78 27.1,15.7 27.61,15.7 28.14,16.23 v28.32,16.23
  Bottom 0.152: v28.32,16.23 28.14,16.23 27.61,15.7 27.1,15.7 27.02,15.78 U3.37
GP183_PWM3  (via drill 0.33)
  Top 0.152: v29.39,16.41 29.39,16.36 28.6,15.57 27.91,15.57 27.74,15.39 26.62,15.39 26.61,15.38 U3.39
  Bottom 0.152: U3.39 26.61,15.38 26.62,15.39 27.74,15.39 27.91,15.57 28.6,15.57 29.39,16.36 v29.39,16.41
MSIC_SLP_CLK  (via drill 0.33)
  Top 0.152: v27.51,21.46 27.19,21.78 U3.7
  Bottom 0.152: U3.7 27.19,21.78 v27.51,21.46
N$1
  Top 0.61: SJ1.2 D1.A
N$2
  Top 0.406: D2.A D4.C 8.81,36.49 R2.1
N$3
  Top 0.152: U1.15 7.38,17.79 11.08,14.09 U4.19
N$4
  Top 0.152: U1.23 12.58,20.83 10.97,19.23 10.97,17.78 11.46,17.29 U4.11
N$5
  Top 0.406: D3.A D5.C 16.17,36.58 R1.1
N$10
  Top 0.152: 9.98,17.4 11.29,16.09 U4.14
  Top 0.178: U1.19 9.98,21.91 9.4,21.34 9.4,20.57 9.98,20 9.98,17.4
N$11
  Top 0.152: U4.17 11.19,14.89 8.38,17.7 8.38,21.61 8.68,21.91 U1.17
N$12
  Top 0.152: U4.18 11.13,14.49 8.03,17.6 U1.16
N$14
  Top 0.152: U1.21 11.28,20.83 10.31,19.86 10.31,17.53 11.34,16.49 U4.13
N$15
  Top 0.152: U1.22 11.93,20.84 10.64,19.56 10.64,17.65 11.4,16.89 U4.12
OSC_CLK_OUT  (via drill 0.33)
  Top 0.152: v27.51,8.33 27.23,8.61 27.23,9.37 26.82,9.78 U3.67
  Bottom 0.152: U3.67 26.82,9.78 27.23,9.37 27.23,8.61 v27.51,8.33
PSW  (via drill 0.33)
  Top 0.152: v29.21,19.53 29.18,19.56 28.17,19.56 27.86,19.25 27.05,19.25 26.78,18.98 U3.21
  Bottom 0.152: U3.21 26.78,18.98 27.05,19.25 27.86,19.25 28.17,19.56 29.18,19.56 v29.21,19.53
PWRBTN#  (via drill 0.33)
  Top 0.152: v28.19,20.52 27.53,19.86 26.8,19.86 26.71,19.78 U3.17
  Bottom 0.152: U3.17 26.71,19.78 26.8,19.86 27.53,19.86 v28.19,20.52
RCVR_MODE  (via drill 0.33)
  Top 0.152: v28.65,17.55 28.12,17.55 27.89,17.32 26.92,17.32 26.58,16.98 U3.31
  Bottom 0.152: U3.31 26.58,16.98 26.92,17.32 27.89,17.32 28.12,17.55 v28.65,17.55
RESET_OUT#  (via drill 0.33)
  Top 0.152: U3.36 22.25,16.18 21.82,15.75 20.5,15.75 v20.27,15.98
  Bottom 0.152: v20.27,15.98 20.5,15.75 21.82,15.75 22.25,16.18 U3.36
USB_DN  (via drill 0.33)
  Top 0.152: U3.18 22.64,19.78 22.5,19.91 19.51,19.91 18.87,20.55 v18.87,21.01
  Bottom 0.152: v18.87,21.01 18.87,20.55 19.51,19.91 22.5,19.91 22.64,19.78 U3.18
USB_DP  (via drill 0.33)
  Top 0.152: v19.79,20.57 20.12,20.24 22.63,20.24 22.7,20.18 U3.16
  Bottom 0.152: U3.16 22.7,20.18 22.63,20.24 20.12,20.24 v19.79,20.57
USB_ID  (via drill 0.33)
  Top 0.152: v27.51,22.86 27.23,22.58 U3.3
  Bottom 0.152: U3.3 27.23,22.58 v27.51,22.86
USB_VBUS  (via drill 0.33)
  Top 0.152: v18.49,19.99 18.87,19.61 22.28,19.61 22.5,19.38 U3.20
  Bottom 0.152: U3.20 22.5,19.38 22.28,19.61 18.87,19.61 v18.49,19.99
V_BAT_BKUP  (via drill 0.33)
  Top 0.152: v28.45,18.87 28.37,18.95 27.18,18.95 26.81,18.58 U3.23
  Bottom 0.152: U3.23 26.81,18.58 27.18,18.95 28.37,18.95 v28.45,18.87
VIN
  Top 0.61: JP2.2 20.7,38.99 19.94,38.23 D1.C 19.94,35.18 15.75,30.99 C1.A 13.23,25.55 13.23,24.41
  pour Top: 5.79,22.1 7.06,22.1 7.06,22.33 7.04,23.72 10.31,23.72 10.31,22.15 10.95,22.15 10.95,23.72 12.9,23.72 12.9,22.15 13.46,22.15 13.46,24.82 5.79,24.82
VSYS  (via drill 0.33, 0.51)
  Top 0.152: U3.6 22.65,22.18 22.48,22.35 22.48,22.84 v22.11,23.21
  Top 0.178: U1.20 10.63,21.3 v10.41,21.08 | v11.05,12.19 C2.1 13.21,13.04 13.21,14.99 12.9,15.29 U4.16
  Top 0.305: SJ1.1 19.94,25.38 v22.11,23.21
  Bottom 0.152: U3.6 22.65,22.18 22.1,22.73 22.1,23.21 v22.11,23.21
  Bottom 0.178: v11.05,12.19 10.41,12.83 v10.41,21.08 12.7,23.37 21.95,23.37 v22.11,23.21
  pour Top (isolate 0.051, rank 2): 22.73,22.1 23.88,22.1 23.88,23.11 22.73,23.11 22.23,23.62 21.97,23.62 21.72,23.37 21.72,22.99 22.61,22.1
  pour Bottom (isolate 0.051, rank 2): 22.73,22.1 23.88,22.1 23.88,23.11 22.73,23.11 22.23,23.62 21.97,23.62 21.72,23.37 21.72,22.99 22.61,22.1

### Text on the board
Top: v10
tPlace: GND | VIN | B1 | B2 | A2 | A1 | Dual H-bridge | VSYS->VIN
bPlace: Dual H-bridge | B1 | B2 | A2 | A1 | GND | VIN | 4xM2.0
tDocu: Note: Units are in Inches | Casey Kuhns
